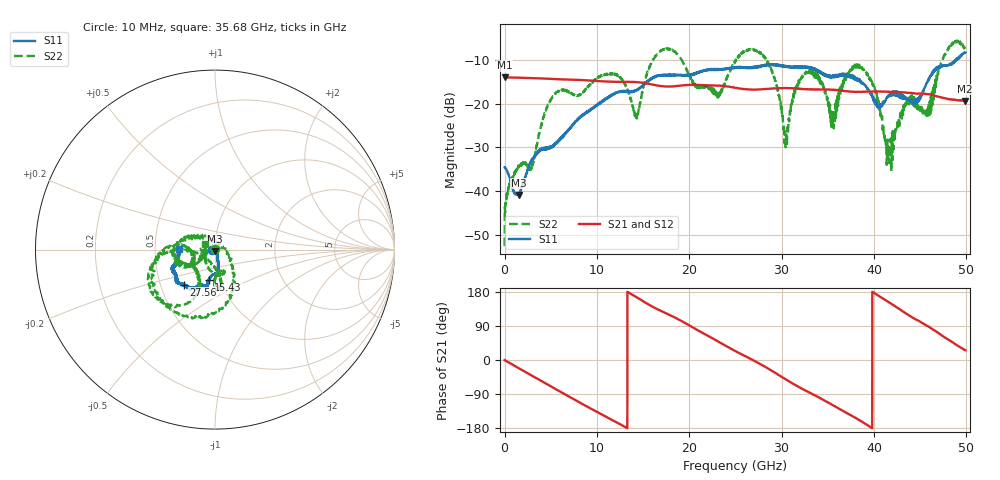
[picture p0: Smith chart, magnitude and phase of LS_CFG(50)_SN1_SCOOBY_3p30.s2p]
!Keysight Technologies,N5245B,MY58422026,A.13.80.08
!Date: Thursday, March 19, 2020 23:42:33
!Correction: S11(Full 2 Port(1,2))
!S21(Full 2 Port(1,2))
!S12(Full 2 Port(1,2))
!S22(Full 2 Port(1,2))
!S2P File: Measurements: S11, S21, S12, S22:
# Hz S DB R 50.0
!freq dBS11 angS11 dBS21 angS21 dBS12 angS12 dBS22 angS22
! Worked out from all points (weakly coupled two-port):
!   4991 points, 10 MHz to 49.91 GHz, reference 50 ohm
!   highest |S21| = -14.00 dB at 10 MHz (marker M1); lowest = -19.4 dB at 49.82 GHz (marker M2)
!   lowest |S11| = -40.9 dB at 1.53 GHz (marker M3), VSWR 1.02, Z = 49.7 - j0.857 ohm
!   |S11| at or under -10 dB: start of sweep to 48.88 GHz; 48.94539 GHz to 48.98359 GHz (38.2 MHz wide, 0.078 % of centre)
!   |S22| runs from -52.6 to -5.6 dB; largest |S21 - S12| = 0.0019
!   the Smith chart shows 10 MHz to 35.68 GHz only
!   S11 on the Smith chart (normalised r, x): 10 MHz: 0.96, -0.01; 15.43 GHz: 0.88, -0.31; 27.56 GHz: 0.66, -0.28; 35.68 GHz: 0.66, +0.00
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1e7  -34.59 -171.3  -14.00 -0.3  -13.98 -0.3  -52.61 157.3
1.53e9  -40.89 -107.4  -14.09 -21.5  -14.08 -21.5  -34.33 -20.7
2.94e9  -32.78 -61.1  -14.19 -41.1  -14.18 -41.0  -34.82 114.4
5.38e9  -29.27 -68.4  -14.39 -74.8  -14.39 -74.8  -18.03 -96.9
8.33e9  -23.01 -75.8  -14.63 -114.8  -14.62 -114.7  -17.72 -81.6
1.205e10  -17.65 -84.8  -15.03 -163.5  -15.03 -163.4  -13.32 -84.4
1.427e10  -16.91 -95.6  -15.10 166.0  -15.09 166.1  -22.88 -129.9
1.543e10  -15.21 -101.5  -15.42 149.0  -15.42 149.1  -13.23 179.7
1.665e10  -13.68 -102.7  -15.91 132.9  -15.90 133.0  -8.45 -162.6
2.301e10  -12.35 -117.9  -15.89 50.5  -15.89 50.7  -18.44 -165.2
2.496e10  -11.84 -122.8  -16.36 23.9  -16.34 24.1  -10.50 -175.4
2.756e10  -11.57 -131.6  -16.79 -8.9  -16.79 -8.6  -8.40 -102.8
3.047e10  -11.61 -144.1  -16.47 -51.2  -16.46 -51.0  -29.20 46.1
3.162e10  -11.50 -150.2  -16.58 -67.7  -16.57 -67.4  -15.96 151.0
3.328e10  -11.90 -158.7  -16.76 -89.4  -16.76 -89.0  -12.67 -164.6
3.568e10  -13.76 179.1  -16.88 -120.7  -16.82 -120.3  -22.97 150.6
3.851e10  -14.87 170.5  -17.34 -160.0  -17.31 -160.2  -11.49 -154.6
4.16e10  -18.09 100.0  -17.31 152.7  -17.33 152.7  -29.96 105.6
4.675e10  -11.79 6.1  -18.31 75.2  -18.33 75.3  -14.05 -140.4
4.841e10  -10.90 -8.1  -19.11 48.6  -19.15 48.6  -6.37 -64.6
4.982e10  -8.40 -17.4  -19.39 26.8  -19.40 26.9  -7.22 -11.8
4.991e10  -8.35 -16.5  -19.37 25.7  -19.39 25.7  -7.83 -12.0
